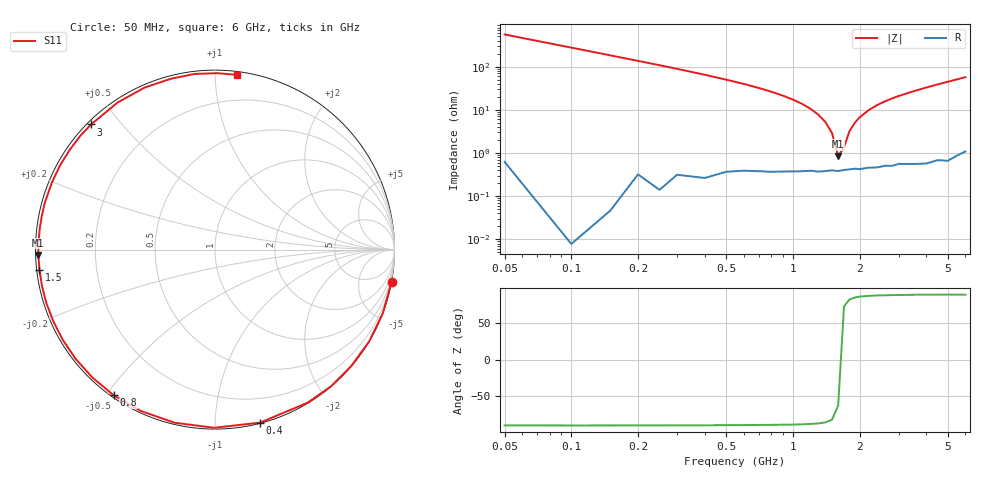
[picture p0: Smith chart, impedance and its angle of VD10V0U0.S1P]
! Infineon Technologies  Discrete & RF Semiconductors
! BBY 55-03
! Si Tuning Diode in SOD323
! VR = 10 V
! S-Parameters:  June  1999
# GHz  S  MA  R  50
!  f  S11
! GHz  MAG  ANG
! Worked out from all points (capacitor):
!   34 points, 50 MHz to 6 GHz, reference 50 ohm
!   read as one part to ground: C = 5.76 pF near 50 MHz
!   lowest |Z| = 834 mohm at 1.6 GHz (marker M1)
!   series resonance near 1.636 GHz, so ESL is about 1.6 nH
!   S11 on the Smith chart (normalised r, x): 50 MHz: 0, -11; 400 MHz: 0.01, -1.29; 800 MHz: 0.01, -0.52; 1.5 GHz: 0.01, -0.06; 3 GHz: 0.01, +0.42; 6 GHz: 0.02, +1.13
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0.05  0.9998 -10.3
0.1  1 -20.6
0.15  0.9999 -30.7
0.2  0.9985 -40.5
0.25  0.999 -49.8
0.3  0.997 -58.8
0.4  0.9961 -75.4
0.5  0.9927 -90.2
0.6  0.9905 -103.1
0.7  0.9893 -114.6
0.8  0.9886 -124.8
0.9  0.9875 -133.9
1  0.9868 -142.0
1.1  0.9861 -149.4
1.3  0.9856 -162.4
1.5  0.9843 -173.4
1.6  0.9849 -178.3
1.8  0.9836 172.7
2  0.9836 164.8
2.4  0.9828 151.2
2.8  0.9824 139.8
3  0.9812 134.7
3.5  0.9829 123.5
4  0.9842 113.4
4.5  0.9831 104.5
5  0.9854 96.6
5.5  0.983 89.2
6  0.9813 82.8
